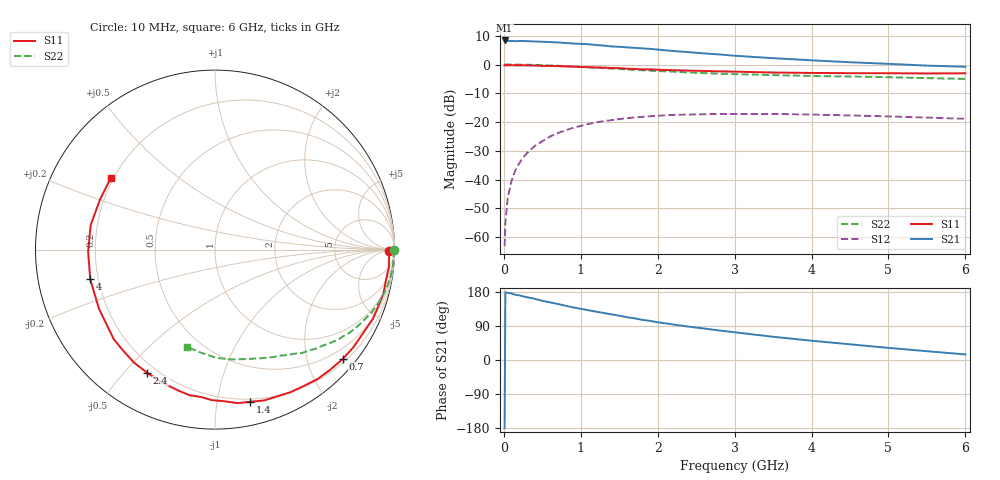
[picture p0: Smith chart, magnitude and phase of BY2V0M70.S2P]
! SIEMENS Small Signal Semiconductors
! BFY420
! Si NPN RF SIEGET Grounded Emitter Transistor in MICRO-X
! VCE = 2 V  IC = 0.7 mA
! Common Emitter S-Parameters:  October  1996
# GHz  S  MA  R  50
!  f  S11  S21  S12  S22
! GHz  MAG  ANG  MAG  ANG  MAG  ANG  MAG  ANG
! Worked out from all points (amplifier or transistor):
!   36 points, 10 MHz to 6 GHz, reference 50 ohm
!   highest |S21| = 8.4 dB at 10 MHz (marker M1)
!   |S21| within 3 dB of that: start of sweep to 1.932 GHz
!   unconditionally stable (mu >= 1): 4.703 GHz to end of sweep
!   at 250 MHz: K = 0.03, MSG = 20.3 dB, |S12| = -32.3 dB
!   at 1.4 GHz: K = 0.18, MSG = 12.8 dB, |S12| = -19.3 dB
!   at 6 GHz: K = 1.37, MAG = 5.4 dB, |S12| = -18.8 dB
!   S11 on the Smith chart (normalised r, x): 10 MHz: 62, -23; 700 MHz: 0.27, -2.69; 1.4 GHz: 0.18, -1.24; 2.4 GHz: 0.16, -0.58; 4 GHz: 0.17, -0.11; 6 GHz: 0.19, +0.30
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0.01  0.9718 -0.6  2.618 -179.3  0.0007 94.4  0.9999 -0.2
0.02  0.9692 -1.5  2.591 178.8  0.0018 95.7  0.9978 -0.5
0.05  0.9713 -3.0  2.562 177.1  0.0048 90.1  0.9987 -1.4
0.1  0.974 -5.8  2.566 175.7  0.0096 88.6  0.9935 -2.9
0.15  0.9687 -9.0  2.545 172.1  0.0145 85.7  0.996 -4.3
0.2  0.9674 -11.9  2.561 170.7  0.0192 83.5  0.9949 -5.7
0.25  0.9701 -14.6  2.569 168.1  0.0242 80.5  0.9925 -7.2
0.4  0.9604 -23.6  2.519 161.6  0.0383 75.5  0.983 -11.4
0.5  0.9474 -29.4  2.483 156.1  0.0466 72.1  0.9739 -14.2
0.7  0.9372 -40.5  2.418 147.9  0.0643 64.6  0.9511 -19.6
0.9  0.9203 -51.5  2.317 138.8  0.0795 57.8  0.9233 -24.5
1.1  0.8986 -62.3  2.252 131.3  0.0927 51.5  0.8948 -29.4
1.4  0.8697 -77.1  2.062 120.4  0.1081 42.7  0.8516 -35.8
1.8  0.8247 -95.5  1.907 106.0  0.1232 32.3  0.7948 -43.2
2.2  0.7972 -111.9  1.716 93.8  0.1333 23.3  0.7524 -50.0
2.4  0.7833 -118.9  1.641 88.1  0.1351 19.8  0.7266 -53.1
2.8  0.7606 -132.4  1.497 77.9  0.1383 12.9  0.6923 -58.7
3.5  0.7257 -152.9  1.289 61.3  0.1387 3.6  0.655 -67.7
4  0.7145 -166.6  1.185 50.9  0.1353 -1.4  0.6333 -74.4
4.5  0.7071 -179.0  1.095 41.4  0.1304 -5.8  0.6187 -81.4
5.5  0.6987 156.8  0.957 23.2  0.1197 -10.0  0.5804 -97.4
6  0.7045 145.6  0.914 14.7  0.1142 -10.0  0.5635 -106.3
